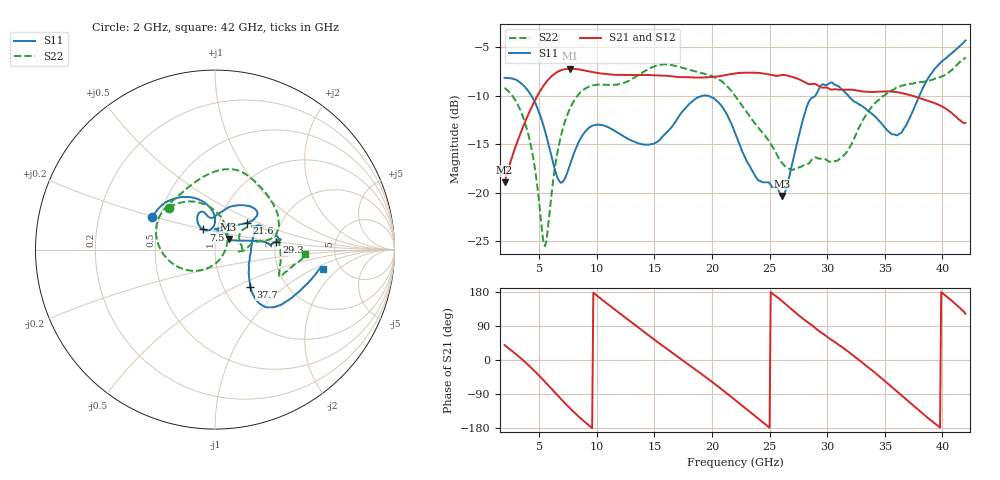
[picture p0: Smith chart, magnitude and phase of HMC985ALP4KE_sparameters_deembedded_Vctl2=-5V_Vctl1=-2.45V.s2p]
!s2p File: Measurements: S11, S21, S12, S22
# GHz S dB R 50.0
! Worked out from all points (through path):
!   401 points, 2 GHz to 42 GHz, reference 50 ohm
!   highest |S21| = -7.20 dB at 7.7 GHz (marker M1); lowest = -18.9 dB at 2 GHz (marker M2)
!   lowest |S11| = -20.3 dB at 26.1 GHz (marker M3), VSWR 1.21, Z = 57.7 + j6.97 ohm
!   |S11| at or under -10 dB: 4.331 GHz to 19.14 GHz (14.81 GHz wide, 126 % of centre); 19.72 GHz to 28.95 GHz (9.229 GHz wide, 37.9 % of centre); 31.85 GHz to 38 GHz (6.149 GHz wide, 17.6 % of centre)
!   |S22| runs from -25.5 to -6.0 dB; largest |S21 - S12| = 0.00054
!   S11 on the Smith chart (normalised r, x): 2 GHz: 0.46, +0.19; 7.5 GHz: 0.86, +0.20; 21.6 GHz: 1.36, +0.43; 29.3 GHz: 2.03, +0.20; 37.7 GHz: 1.34, -0.61; 42 GHz: 3.67, -1.26
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2  -8.14 152.8  -18.92 39.3  -18.93 39.3  -9.17 137.9
4  -9.42 119.8  -12.05 -11.6  -12.06 -11.6  -13.71 86.8
5.5  -13.60 93.0  -8.75 -57.6  -8.76 -57.6  -25.50 -31.3
6.7  -18.71 100.5  -7.46 -97.0  -7.46 -97.0  -15.14 -137.8
7.5  -17.71 120.5  -7.20 -122.2  -7.21 -122.2  -11.79 -164.6
7.7  -17.01 122.5  -7.20 -128.3  -7.20 -128.2  -11.24 -170.1
8.7  -14.18 120.5  -7.33 -156.5  -7.33 -156.5  -9.51 167.6
10.4  -13.00 109.1  -7.69 160.6  -7.70 160.6  -8.84 142.9
12.4  -14.20 103.1  -7.85 113.7  -7.85 113.7  -8.64 118.0
15.4  -14.61 89.4  -7.91 44.6  -7.91 44.6  -6.83 79.8
18.3  -10.56 56.2  -8.10 -19.4  -8.10 -19.4  -7.39 51.4
21.6  -12.66 39.8  -7.76 -95.6  -7.77 -95.6  -9.37 12.7
22  -13.78 43.8  -7.69 -105.4  -7.69 -105.4  -9.98 10.9
24.1  -18.76 86.3  -7.63 -156.7  -7.64 -156.6  -13.40 9.9
26.1  -20.33 38.4  -7.83 155.1  -7.84 155.2  -16.94 -3.6
28.7  -10.17 4.3  -8.78 91.3  -8.78 91.4  -16.52 1.9
29.3  -9.24 7.2  -9.02 76.2  -9.02 76.3  -16.48 3.7
32.5  -10.67 25.8  -9.43 6.2  -9.43 6.2  -13.97 35.5
35.4  -13.74 6.6  -9.54 -65.7  -9.55 -65.7  -9.61 15.0
37.7  -10.84 -46.5  -10.09 -126.3  -10.09 -126.2  -8.66 -6.1
39.7  -6.74 -44.1  -10.92 -176.0  -10.92 -175.9  -8.12 -22.4
42  -4.28 -10.2  -12.78 121.9  -12.79 122.0  -6.03 -2.8
